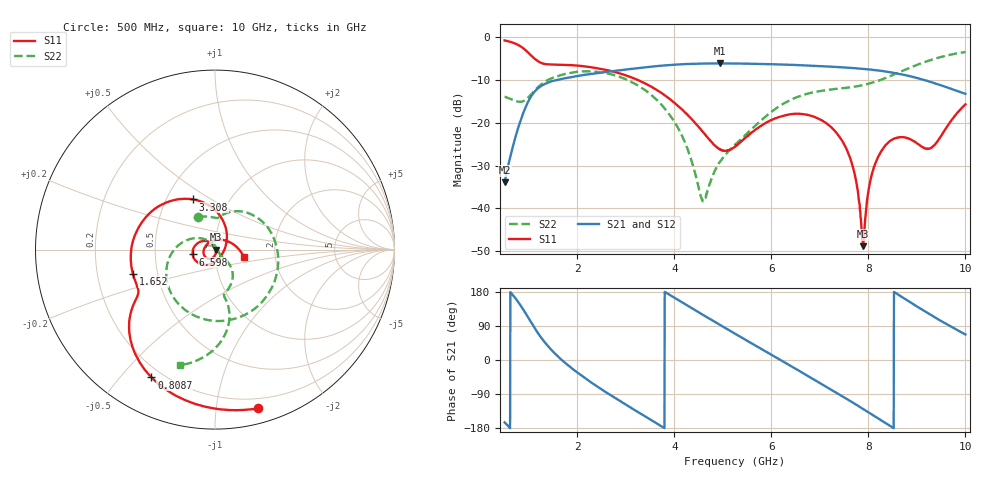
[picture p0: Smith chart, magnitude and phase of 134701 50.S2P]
!  2-Port S-parameters saved by WinCal
! VAR MeasName=S-Parameters (CALIBRATED_DATA) read from VNA (N5242A)
! VAR MeasDate=2013-7-3 16:39:32
! VAR NAME=134701 50
! VAR FILENAME=134701 50.S2P
! VAR DATE=2013-7-3 16:39:32
! VAR PHYS_PORTS=1,2
# Hz S MA R 50
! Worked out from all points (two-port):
!   1601 points, 500 MHz to 10 GHz, reference 50 ohm
!   highest |S21| = -6.11 dB at 4.947 GHz (marker M1); lowest = -33.9 dB at 500 MHz (marker M2)
!   |S21| within 3 dB of the highest: 1.977 GHz to 8.859 GHz (6.882 GHz wide, 127 % of centre)
!   lowest |S11| = -48.8 dB at 7.892 GHz (marker M3), VSWR 1.01, Z = 50.4 + j0.0387 ohm
!   |S11| at or under -10 dB: 3.251 GHz to end of sweep
!   |S22| runs from -38.3 to -3.4 dB; largest |S21 - S12| = 0.002
!   S11 on the Smith chart (normalised r, x): 500 MHz: 0.12, -1.30; 808.8 MHz: 0.16, -0.61; 1.652 GHz: 0.36, -0.13; 3.308 GHz: 0.68, +0.42; 6.598 GHz: 0.78, -0.04; 10 GHz: 1.37, -0.11
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5e8  0.917 -74.8  0.0203 -164.6  0.02026 -164.9  0.202 117.3
8.0875e8  0.7952 -116.4  0.09867 147.8  0.09853 147.7  0.1761 88.1
1.200625e9  0.5189 -147.9  0.2571 68.6  0.2571 68.5  0.2653 52.5
1.651875e9  0.4772 -163.4  0.3241 3.1  0.3242 3.0  0.3601 -12.0
2.085312e9  0.4616 175.5  0.3589 -41.2  0.3583 -41.4  0.3988 -63.0
2.750312e9  0.3959 142.4  0.4031 -98.1  0.4018 -98.2  0.3621 -125.6
3.308438e9  0.3055 113.7  0.4398 -141.9  0.4388 -141.9  0.2606 -169.1
3.670625e9  0.2358 94.1  0.4624 -170.0  0.4612 -170.0  0.1776 164.9
4.193125e9  0.1373 64.3  0.4844 149.5  0.4841 149.6  0.06368 127.3
4.579062e9  0.07957 35.6  0.4923 119.9  0.4924 119.9  0.01264 39.3
4.947188e9  0.04875 -12.7  0.4948 92.0  0.4947 92.1  0.03556 -42.5
5.25e9  0.05249 -62.9  0.4929 69.4  0.4935 69.4  0.05587 -46.4
5.944688e9  0.1044 -125.1  0.4849 17.9  0.4849 17.9  0.127 -47.2
6.597812e9  0.1272 -167.7  0.471 -30.5  0.4712 -30.7  0.2065 -63.4
6.835312e9  0.1204 176.8  0.4648 -48.3  0.4648 -48.3  0.2253 -69.4
7.559688e9  0.04781 122.9  0.4412 -103.2  0.4415 -103.2  0.2579 -78.7
7.737812e9  0.02219 103.7  0.4338 -117.1  0.4339 -117.2  0.2659 -78.8
7.892188e9  0.003631 6.1  0.4271 -129.1  0.4266 -129.2  0.2764 -78.3
8.088125e9  0.02708 -85.9  0.4162 -144.8  0.4164 -144.8  0.2961 -77.4
8.420625e9  0.05971 -120.3  0.3927 -171.7  0.3923 -171.9  0.3457 -77.0
9.281562e9  0.05064 100.4  0.3006 119.3  0.3002 119.1  0.5418 -89.1
1e10  0.1646 -14.1  0.2183 67.5  0.2174 67.4  0.6724 -106.9
